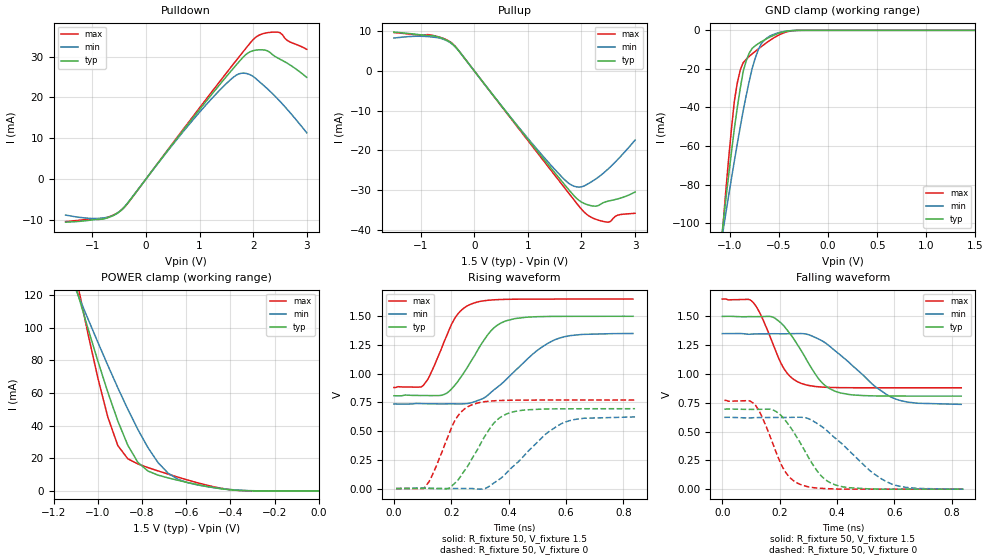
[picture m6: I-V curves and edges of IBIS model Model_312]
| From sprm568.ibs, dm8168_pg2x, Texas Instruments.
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| Model based on original model for BSHTLTCSCDDVGPBFZ
|   Sub model FAST_7MA_10PER_P_1P5
[model]   Model_312
|[Description]  [1.5V-3-STATE-X-FAST:7MA, IND, 10%]
|   Fast slew rate (SR[1:0] = "10"), 1.14 * RExt = 0.875 * Iout
|   (I[2:0] = "010"), 7mA nominal with Rext = 50R, ,Industrial
|   temperature range (-40C to 125C, 25C nominal),10% power supply
|   tolerance
|[Input Load]
|[Output Drive] FAST:7MA
|Voltage   1.5V
|Mode   3-STATE
Model_type   3-state
Polarity   Non-Inverting
Enable   Active-Low
Cref =  15.0000pF
Rref =  100.0000M
Vref =  0V
Vmeas =  0.75
C_comp   1.5249p   1.4275p   1.6205p
[Model Spec]
[Temperature Range]   25   125   -40
[Voltage Range]   1.5   1.35   1.65
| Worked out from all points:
|   slope of the pulldown table from 0 to 0.225 V, typ, clamps not added: 57.5 ohm
|   slope of the pullup table from 0 to 0.225 V, typ, clamps not added: 57.5 ohm
|   GND clamp passes 1 mA (typ) near -0.47 V on its own axis
|   POWER clamp passes 1 mA (typ) near -0.42 V on its own axis
|   rising waveform, R_fixture 50, V_fixture 1.5: 20-80 % time 108ps typ, 165ps min, 81.9ps max; typ from 0.808 V to 1.5 V
|   rising waveform, R_fixture 50, V_fixture 0: 20-80 % time 103ps typ, 154ps min, 78.5ps max; typ from 0 V to 0.695 V
|   falling waveform, R_fixture 50, V_fixture 1.5: 20-80 % time 108ps typ, 170ps min, 81.1ps max; typ from 1.5 V to 0.807 V
|   falling waveform, R_fixture 50, V_fixture 0: 20-80 % time 104ps typ, 165ps min, 78.5ps max; typ from 0.694 V to 0 V
[POWER_clamp]
-1.5V     321.6mA    260.6mA    415.8mA
-1.091V   121.1mA    120.8mA    126.6mA
-1.076V   114.1mA    115.8mA    116.8mA
-1V       79.88mA    91.3mA     69.56mA
-954.5mV  60.58mA    77.05mA    45.34mA
-909.1mV  42.84mA    63.2mA     27.8mA
-818.2mV  17.47mA    37.6mA     16.51mA
-772.7mV  12.19mA    26.53mA    14.33mA
-681.8mV  7.985mA    10.89mA    10.33mA
-590.9mV  5.092mA    4.952mA    6.596mA
-363.6mV  298.9uA    465.6uA    298.1uA
0V        1.518nA    23.05nA    396.5pA
[Pulldown]
-1.5V     -10.59mA   -8.84mA    -10.44mA
-772.7mV  -9.742mA   -9.502mA   -9.607mA
-590.9mV  -8.819mA   -8.812mA   -8.723mA
-409.1mV  -6.984mA   -6.933mA   -7.018mA
954.5mV   16.28mA    15.69mA    16.68mA
1.455V    24.41mA    22.83mA    25.23mA
1.727V    28.63mA    25.76mA    29.8mA
2V        31.49mA    25.17mA    34.2mA
2.318V    31.02mA    21.5mA     35.98mA
2.5V      29.41mA    19.07mA    35.92mA
2.636V    28.42mA    17.09mA    34mA
3V        24.94mA    11.34mA    31.82mA
[Pullup]
-1.5V     9.77mA     8.27mA     9.66mA
-818.2mV  8.911mA    8.576mA    9.063mA
-409.1mV  6.818mA    6.713mA    6.907mA
1.227V    -21.03mA   -20.59mA   -21.46mA
1.682V    -28.55mA   -27.31mA   -29.35mA
1.864V    -31.44mA   -29.02mA   -32.49mA
2V        -32.99mA   -29.17mA   -34.79mA
2.182V    -33.9mA    -27.92mA   -36.81mA
2.409V    -33.14mA   -25.72mA   -37.87mA
2.545V    -32.62mA   -24.06mA   -37.83mA
2.682V    -32.18mA   -22.2mA    -36.26mA
3V        -30.46mA   -17.41mA   -35.81mA
[GND_clamp]
-1.5V     -310mA     -250.5mA   -402.4mA
-1.076V   -103.5mA   -106.1mA   -105.2mA
-1.045V   -89.74mA   -96.32mA   -85.93mA
-954.5mV  -51.19mA   -67.85mA   -36.85mA
-924.2mV  -40.06mA   -58.84mA   -27.27mA
-863.6mV  -21.23mA   -41.55mA   -16.73mA
-833.3mV  -15.79mA   -33.74mA   -15.03mA
-772.7mV  -9.342mA   -19.74mA   -12.19mA
-712.1mV  -6.927mA   -10.35mA   -9.702mA
-621.2mV  -4.26mA    -3.894mA   -6.224mA
-409.1mV  -336.9uA   -288.9uA   -618.6uA
1.5V      1.518nA    2.298uA    269.6pA
[Ramp]
dV/dt_f   0.554192/0.16199054n   0.49156/0.24375116n   0.616528/0.1254695n
dV/dt_r 0.55902384/0.1539764n 0.50325856/0.22702867n 0.61757096/0.12068165n
R_load = 50
[Rising Waveform]
R_fixture = 50
V_fixture = 1.5
V_fixture_min = 1.35
V_fixture_max = 1.65
0s        808mV      736.6mV    880.1mV
102.4ps   810.4mV    738.9mV    899mV
188.6ps   838.4mV    737.9mV    1.358V
225.4ps   941.6mV    737.2mV    1.528V
272.3ps   1.122V     749.2mV    1.609V
332.3ps   1.355V     823.4mV    1.64V
391.2ps   1.461V     949.5mV    1.647V
497.2ps   1.496V     1.198V     1.65V
576.6ps   1.499V     1.31V      1.65V
833.3ps   1.5V       1.35V      1.65V
[Rising Waveform]
R_fixture = 50
V_fixture = 0
V_fixture_min = 0
V_fixture_max = 0
7.45ps    0V         0V         0V
108.2ps   2.917mV    2.783mV    12.93mV
128.3ps   0V         2.513mV    86.59mV
193.3ps   4.977mV    0V         481.8mV
224.8ps   79.01mV    0V         638.1mV
272.7ps   262.7mV    0V         730.1mV
347.6ps   566.9mV    46.58mV    763.9mV
404.1ps   659.7mV    165.9mV    768.9mV
586.5ps   694.4mV    567.6mV    770.8mV
840.8ps   695.2mV    623.8mV    770.9mV
[Falling Waveform]
R_fixture = 50
V_fixture = 1.5
V_fixture_min = 1.35
V_fixture_max = 1.65
0s        1.499V     1.35V      1.649V
105.9ps   1.497V     1.346V     1.625V
174.8ps   1.494V     1.349V     1.273V
214.5ps   1.418V     1.348V     1.049V
275.4ps   1.202V     1.35V      917.5mV
342.4ps   938.8mV    1.294V     887.1mV
411.1ps   835.5mV    1.165V     880.9mV
529ps     809.4mV    899mV      879.7mV
603.5ps   807.7mV    783.1mV    879.6mV
833.3ps   807.4mV    735.7mV    879.4mV
[Falling Waveform]
R_fixture = 50
V_fixture = 0
V_fixture_min = 0
V_fixture_max = 0
7.45ps    694.3mV    623.1mV    770.3mV
113.6ps   691.7mV    620.5mV    735.2mV
172.1ps   691.6mV    622.2mV    423.1mV
214.3ps   613.7mV    621.7mV    173.4mV
277.7ps   377.3mV    623.4mV    35.39mV
343.9ps   118.4mV    548.6mV    7.275mV
407.8ps   27.17mV    413.7mV    0V
520.8ps   2.344mV    148.8mV    0V
590.2ps   0V         45.13mV    0V
840.8ps   0V         0V         0V
